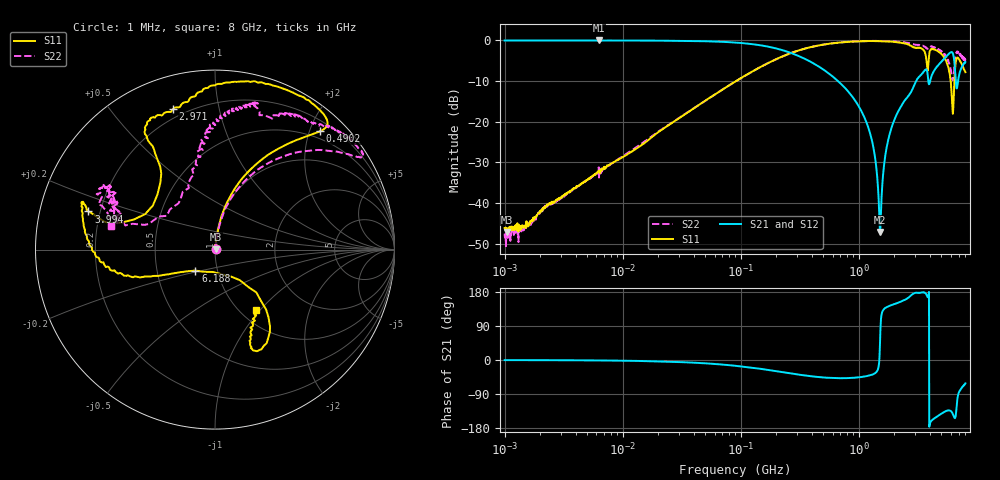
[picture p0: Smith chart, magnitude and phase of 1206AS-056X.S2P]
!s-Parameter Generated by FASTRON Sdn. Bhd.
!FASTRON P/N : 1206AS-056X
!Keysight Technologies: E5071C_MY46733604_B.14.02
!Date: Wed Nov 15 10:21:42 2023
!Version  :Rev00  Wed Nov 15 10:21:42 2023
!Data & Calibration Information:
!Freq  S11:SOLT2(ON)  S21:SOLT2(ON)  S12:SOLT2(ON)  S22:SOLT2(ON)
!PortZ  Port1:50+j0  Port2:50+j0
!When reading reference impedance value at option line is always used.
! Remarks : This data is being provided solely for informational purposes.
# Hz S dB R 50
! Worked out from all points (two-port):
!   1601 points, 1 MHz to 8 GHz, reference 50 ohm
!   highest |S21| = -0.03 dB at 6.301 MHz (marker M1); lowest = -47.1 dB at 1.512 GHz (marker M2)
!   |S21| within 3 dB of the highest: start of sweep to 262.2 MHz; 5.948 GHz to 6.219 GHz (270.3 MHz wide, 4.44 % of centre)
!   lowest |S11| = -47.1 dB at 1.053 MHz (marker M3), VSWR 1.01, Z = 50.4 + j0.139 ohm
!   |S11| at or under -10 dB: start of sweep to 91.17 MHz; 5.997 GHz to 6.448 GHz (451.4 MHz wide, 7.25 % of centre)
!   |S22| runs from -50.6 to -0.1 dB; largest |S21 - S12| = 0.0059
!   S11 on the Smith chart (normalised r, x): 1 MHz: 1.01, +0.00; 490.2 MHz: 0.37, +2.17; 2.971 GHz: 0.16, +0.73; 3.994 GHz: 0.16, +0.14; 6.188 GHz: 0.78, -0.19; 8 GHz: 1.18, -0.95
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1000000  -46.12 16.9  -0.03 -0.3  -0.05 -0.3  -47.49 21.2
1052806  -47.09 18.2  -0.03 -0.3  -0.05 -0.3  -47.70 13.9
4479405  -35.13 74.3  -0.04 -0.9  -0.05 -0.9  -35.30 76.6
6301378  -32.39 71.6  -0.03 -1.2  -0.07 -1.3  -33.70 78.4
2.00676e7  -22.54 81.9  -0.08 -3.7  -0.09 -3.6  -22.43 81.3
8.994653e7  -10.10 73.9  -0.54 -15.2  -0.54 -15.2  -10.14 72.0
4.006501e8  -1.60 50.2  -5.43 -43.1  -5.43 -43.1  -1.61 41.6
4.901632e8  -1.09 48.4  -6.97 -45.9  -6.98 -45.9  -1.09 37.9
1.1258e9  -0.20 56.0  -19.17 -43.4  -19.18 -43.5  -0.19 32.5
1.341815e9  -0.19 61.1  -26.96 -36.8  -26.97 -36.8  -0.17 33.6
1.511962e9  -0.21 65.5  -47.07 41.7  -47.17 41.9  -0.17 35.0
1.7949e9  -0.31 73.1  -23.88 142.0  -23.90 141.8  -0.22 37.9
2.971081e9  -1.76 106.7  -10.87 176.5  -10.91 176.4  -1.02 52.9
3.548043e9  -2.47 121.2  -7.65 178.1  -7.68 178.1  -1.48 62.0
3.750732e9  -5.15 123.5  -7.17 171.8  -7.18 171.8  -1.98 66.4
3.993958e9  -2.66 163.2  -10.41 -169.6  -10.41 -169.6  -1.42 73.8
5.136407e9  -3.71 -176.1  -4.93 -139.3  -4.89 -139.6  -2.86 90.1
5.696244e9  -6.34 -161.3  -3.51 -133.2  -3.49 -133.5  -5.06 97.0
6.187922e9  -15.92 -133.2  -2.94 -139.3  -2.91 -139.7  -9.49 125.4
6.57347e9  -6.34 -51.8  -8.24 -151.6  -8.22 -152.1  -4.16 162.8
6.959019e9  -4.40 -69.0  -9.73 -90.2  -9.72 -90.9  -2.87 149.9
8e9  -7.81 -55.7  -5.35 -61.7  -5.33 -62.3  -4.54 167.2
